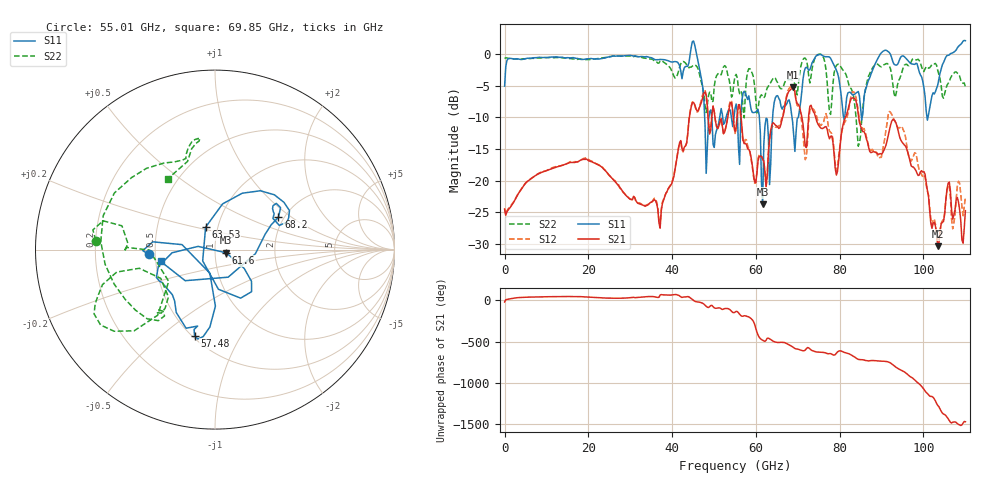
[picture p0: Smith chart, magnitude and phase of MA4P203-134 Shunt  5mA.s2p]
!Keysight Technologies,N5247B,US61255204,A.15.70.20
!Date: Friday, October 21, 2022 15:22:11
!Correction: S11(C  4-Port  )
!S31(C  4-Port  )
!S13(C  4-Port  )
!S33(C  4-Port  )
!S2P File: Measurements: S11, S31, S13, S33:
# Hz S  dB  R 50
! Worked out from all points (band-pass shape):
!   401 points, 10 MHz to 110 GHz, reference 50 ohm
!   highest |S21| = -5.26 dB at 68.75 GHz (marker M1); lowest = -30.3 dB at 103.4 GHz (marker M2)
!   |S21| within 3 dB of the highest: 66.92 GHz to 70.36 GHz (3.445 GHz wide, 5.02 % of centre); 82.17 GHz to 84.16 GHz (1.993 GHz wide, 2.4 % of centre)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
!   lowest |S11| = -23.7 dB at 61.6 GHz (marker M3), VSWR 1.14, Z = 56.6 - j2.03 ohm
!   |S11| at or under -10 dB: 49.44 GHz to 51.36 GHz (1.915 GHz wide, 3.8 % of centre); 60.82 GHz to 63.99 GHz (3.172 GHz wide, 5.08 % of centre); 68.61 GHz to 70.14 GHz (1.522 GHz wide, 2.19 % of centre)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
!   |S22| runs from -14.6 to 0.0 dB; largest |S21 - S12| = 0.17
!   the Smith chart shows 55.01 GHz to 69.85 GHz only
!   S11 on the Smith chart (normalised r, x): 55.01 GHz: 0.46, -0.03; 57.48 GHz: 0.51, -0.65; 61.6 GHz: 1.13, -0.04; 63.53 GHz: 0.87, +0.22; 68.2 GHz: 1.87, +0.80; 69.85 GHz: 0.53, -0.08
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1e7  -5.09 -178.5  -24.47 -19.5  -24.40 -19.1  -0.74 -178.7
1.843332e10  -0.89 145.7  -16.68 43.8  -16.66 43.7  -0.85 145.3
3.685665e10  -0.91 154.5  -26.67 37.9  -26.28 38.5  -1.46 154.3
4.51059e10  2.02 85.1  -7.67 -0.7  -7.62 -2.8  -1.78 115.3
4.813062e10  -18.84 60.0  -6.58 -71.6  -6.41 -72.0  -9.25 113.3
5.5005e10  -8.62 -175.8  -12.29 -142.6  -12.55 -144.1  -3.52 175.6
5.747978e10  -6.13 -103.3  -14.11 172.7  -13.49 178.1  -6.27 -131.1
6.16044e10  -23.74 -15.9  -16.56 -122.8  -16.64 -120.8  -6.75 -132.9
6.352922e10  -17.35 112.6  -12.04 -113.6  -12.41 -110.5  -4.52 -161.2
6.82038e10  -8.02 27.1  -5.69 173.3  -5.23 170.3  -4.02 98.1
6.875375e10  -10.70 16.9  -5.26 157.7  -4.99 153.8  -4.27 98.3
6.985365e10  -10.17 -167.8  -7.86 131.2  -8.14 130.9  -6.48 123.6
7.342832e10  -1.38 178.2  -8.69 112.1  -8.67 107.6  -2.24 156.3
7.645305e10  -0.44 -165.6  -11.53 87.0  -9.93 118.9  -1.30 148.0
7.947778e10  -3.02 -147.6  -18.50 96.4  -17.70 94.9  -1.67 -137.2
8.415235e10  -6.06 -39.1  -8.20 12.8  -7.74 17.8  -12.31 -170.5
8.745205e10  -3.21 49.8  -15.57 -8.5  -15.20 5.2  -2.70 53.5
9.185165e10  0.20 88.6  -12.04 -30.6  -9.08 -23.0  -1.92 76.1
9.817608e10  -1.49 175.9  -18.40 104.7  -15.71 103.8  -0.95 -174.5
1.034006e11  -4.90 -37.5  -30.32 169.0  -30.27 173.6  -2.60 -110.8
1.069753e11  0.16 10.4  -26.06 -34.2  -27.58 -37.7  -3.30 -23.4
1.1e11  2.08 46.1  -24.73 -28.9  -22.58 -27.9  -5.20 10.5
